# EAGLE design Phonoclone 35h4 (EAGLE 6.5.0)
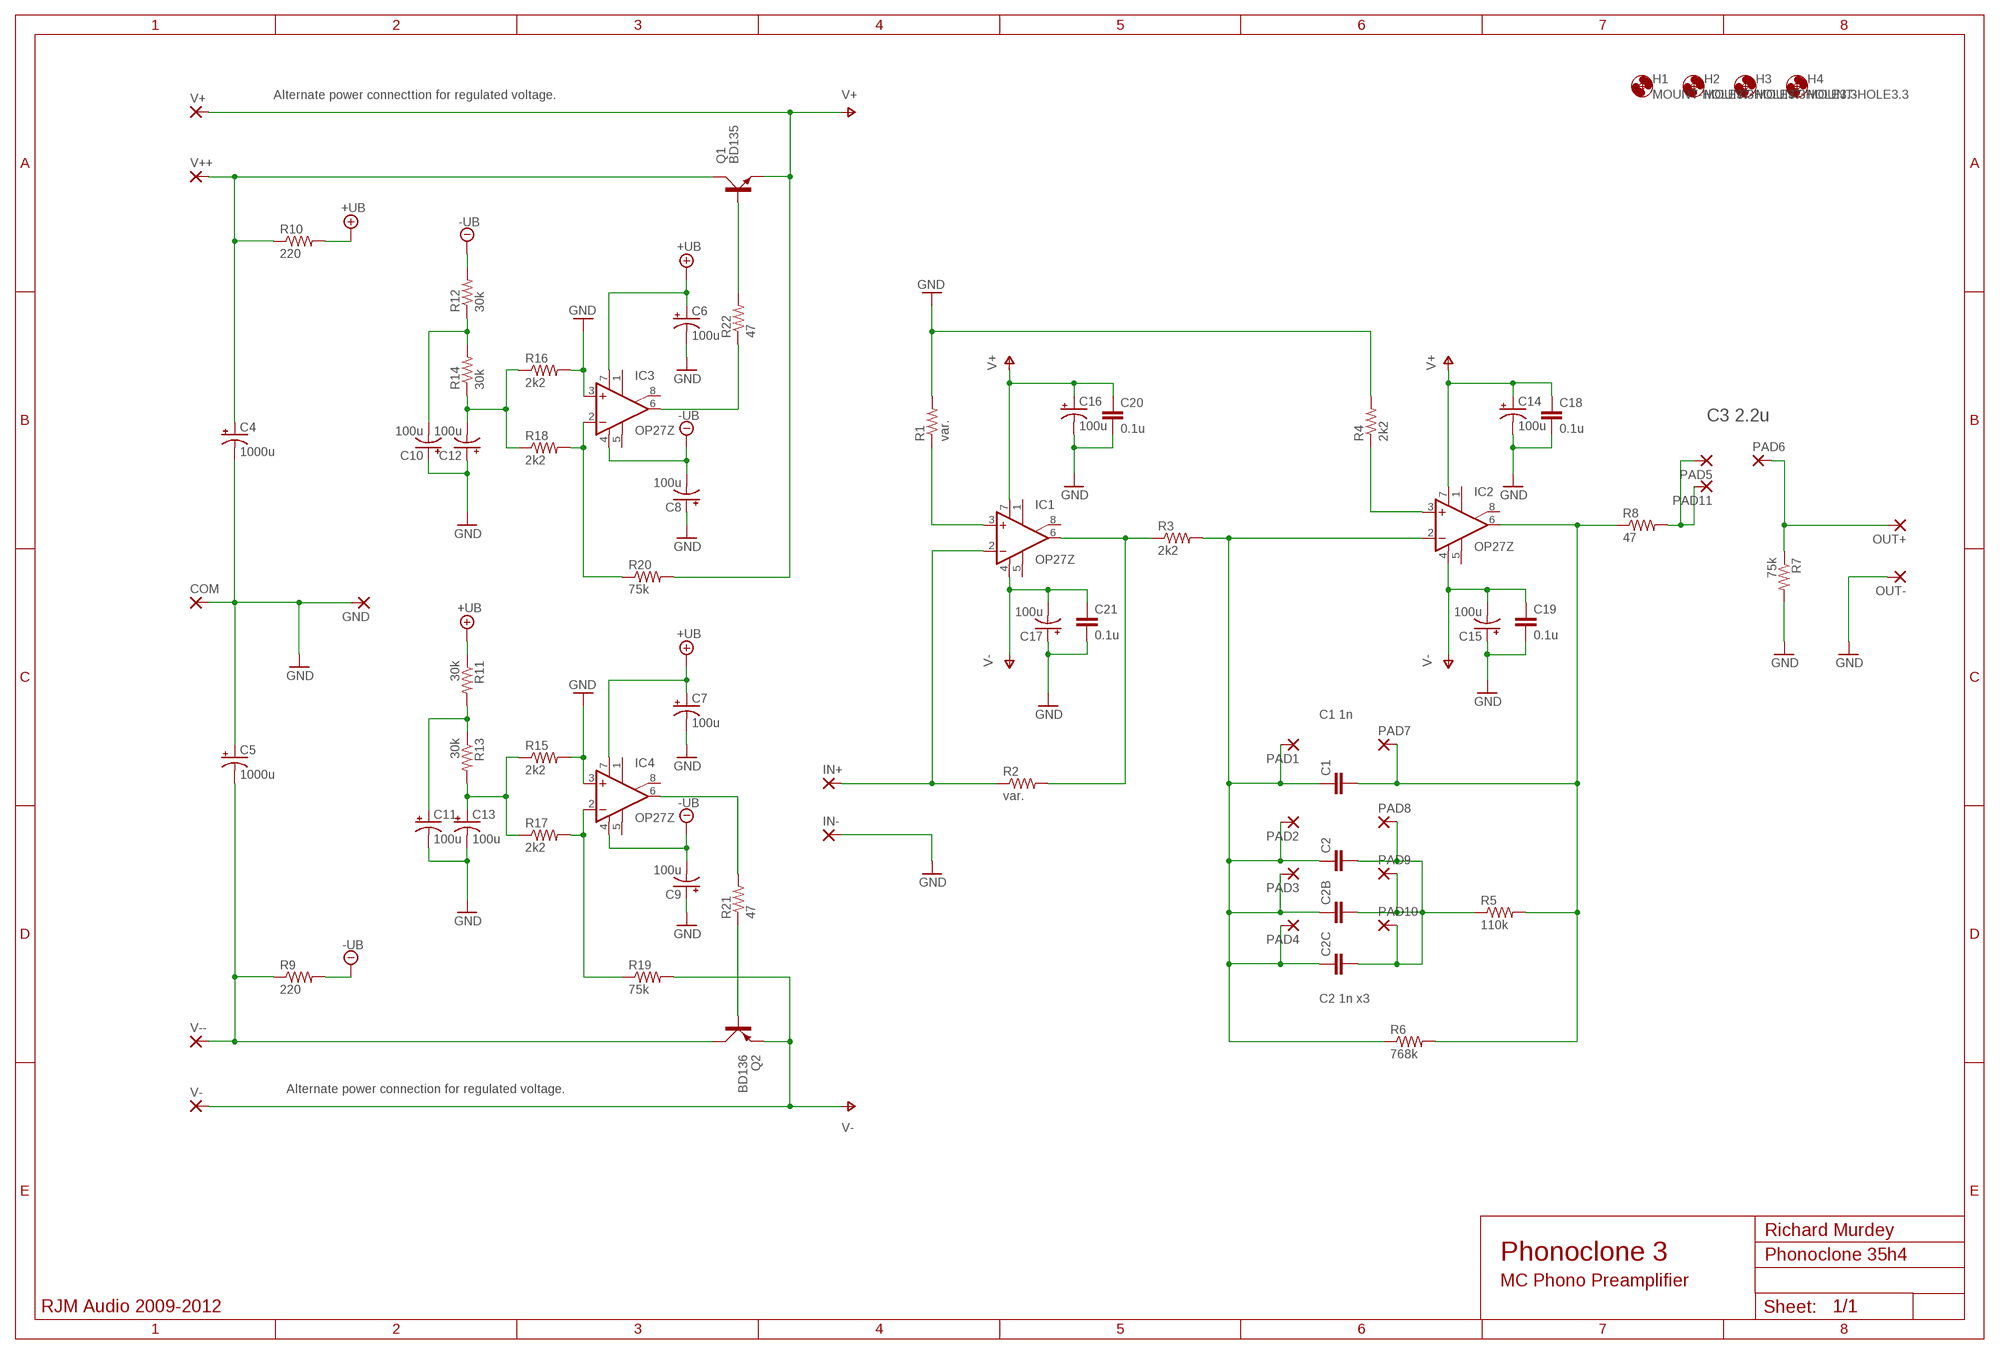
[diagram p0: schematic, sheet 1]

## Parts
C1  C5/4.5  [C5B4.5]
C2  C5/4.5  [C5B4.5]
C2B  C5/4.5  [C5B4.5]
C2C  C5/4.5  [C5B4.5]
C4  1000u  CPOL-USE5-10.5  [E5-10,5]
C5  1000u  CPOL-USE5-10.5  [E5-10,5]
C6  100u  CPOL-USE2.5-6  [E2,5-6]
C7  100u  CPOL-USE2.5-6  [E2,5-6]
C8  100u  CPOL-USE2.5-6  [E2,5-6]
C9  100u  CPOL-USE2.5-6  [E2,5-6]
C10  100u  CPOL-USE2.5-6  [E2,5-6]
C11  100u  CPOL-USE2.5-6  [E2,5-6]
C12  100u  CPOL-USE2.5-6  [E2,5-6]
C13  100u  CPOL-USE2.5-6  [E2,5-6]
C14  100u  CPOL-USE2.5-6  [E2,5-6]
C15  100u  CPOL-USE2.5-6  [E2,5-6]
C16  100u  CPOL-USE2.5-6  [E2,5-6]
C17  100u  CPOL-USE2.5-6  [E2,5-6]
C18  0.1u  C-EU050-024X044  [C050-024X044]
C19  0.1u  C-EU050-024X044  [C050-024X044]
C20  0.1u  C-EU050-024X044  [C050-024X044]
C21  0.1u  C-EU050-024X044  [C050-024X044]
COM  3,17/1,3  [3,17/1,3]
GND  3,17/1,3  [3,17/1,3]
H1  MOUNT-HOLE3.3  [3,3]
H2  MOUNT-HOLE3.3  [3,3]
H3  MOUNT-HOLE3.3  [3,3]
H4  MOUNT-HOLE3.3  [3,3]
IC1  OP27Z  [DIL08]
IC2  OP27Z  [DIL08]
IC3  OP27Z  [DIL08]
IC4  OP27Z  [DIL08]
IN+  2,54/1,1  [2,54/1,1]
IN-  2,54/1,1  [2,54/1,1]
OUT+  2,54/1,1  [2,54/1,1]
OUT-  2,54/1,1  [2,54/1,1]
PAD1  2,54/1,1  [2,54/1,1]
PAD2  2,54/1,1  [2,54/1,1]
PAD3  2,54/1,1  [2,54/1,1]
PAD4  2,54/1,1  [2,54/1,1]
PAD5  2,54/1,1  [2,54/1,1]
PAD6  2,54/1,1  [2,54/1,1]
PAD7  2,54/1,1  [2,54/1,1]
PAD8  2,54/1,1  [2,54/1,1]
PAD9  2,54/1,1  [2,54/1,1]
PAD10  2,54/1,1  [2,54/1,1]
PAD11  2,54/1,1  [2,54/1,1]
Q1  BD135  BD139  [TO126AV]
Q2  BD136  BD140  [TO126AV]
R1  var.  R-US_0207/10  [0207/10]
R2  var.  R-US_0207/10  [0207/10]
R3  2k2  R-US_0207/10  [0207/10]
R4  2k2  R-US_0207/10  [0207/10]
R5  110k  R-US_0207/10  [0207/10]
R6  768k  R-US_0207/10  [0207/10]
R7  75k  R-US_0207/10  [0207/10]
R8  47  R-US_0207/10  [0207/10]
R9  220  R-US_0207/10  [0207/10]
R10  220  R-US_0207/10  [0207/10]
R11  30k  R-US_0207/10  [0207/10]
R12  30k  R-US_0207/10  [0207/10]
R13  30k  R-US_0207/10  [0207/10]
R14  30k  R-US_0207/10  [0207/10]
R15  2k2  R-US_0207/10  [0207/10]
R16  2k2  R-US_0207/10  [0207/10]
R17  2k2  R-US_0207/10  [0207/10]
R18  2k2  R-US_0207/10  [0207/10]
R19  75k  R-US_0207/10  [0207/10]
R20  75k  R-US_0207/10  [0207/10]
R21  47  R-US_0207/10  [0207/10]
R22  47  R-US_0207/10  [0207/10]
V+  3,17/1,3  [3,17/1,3]
V++  3,17/1,3  [3,17/1,3]
V-  3,17/1,3  [3,17/1,3]
V--  3,17/1,3  [3,17/1,3]

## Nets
+UB: C6.+ C7.+ IC3.7(V+) IC4.7(V+) R10.2 R11.1
-UB: C8.- C9.- IC3.4(V-) IC4.4(V-) R9.2 R12.2
GND: C4.- C5.+ C6.- C7.- C8.+ C9.+ C10.+ C11.- C12.+ C13.- C14.- C15.+ C16.- C17.+ C18.2 C19.2 C20.2 C21.2 COM.1(P) GND.1(P) IC3.3(+IN) IC4.3(+IN) IN-.1(P) OUT-.1(P) R1.2 R4.2 R7.2 R15.2 R16.2
IN: IC1.2(-IN) IN+.1(P) R2.1
N$1: PAD5.1(P) PAD11.1(P) R8.2
N$4: C11.+ R11.2 R13.1
N$6: IC3.6(OUT) R22.1
N$7: Q1.B R22.2
N$8: IC1.3(+IN) R1.1
N$9: IC4.2(-IN) R17.2 R19.1
N$10: Q2.B R21.1
N$11: IC4.6(OUT) R21.2
N$13: IC3.2(-IN) R18.2 R20.1
N$14: C10.- R12.1 R14.2
OUT: IC1.6(OUT) R2.2 R3.1
OUT1: C1.2 IC2.6(OUT) PAD7.1(P) R5.2 R6.2 R8.1
OUT2: OUT+.1(P) PAD6.1(P) R7.1
P2+: IC2.3(+IN) R4.1
RIAA1: C1.1 C2.1 C2B.1 C2C.1 IC2.2(-IN) PAD1.1(P) PAD2.1(P) PAD3.1(P) PAD4.1(P) R3.2 R6.1
RIAA2: C2.2 C2B.2 C2C.2 PAD8.1(P) PAD9.1(P) PAD10.1(P) R5.1
V+: C14.+ C16.+ C18.1 C20.1 IC1.7(V+) IC2.7(V+) Q1.E R20.2 V+.1(P)
V++: C4.+ Q1.C R10.1 V++.1(P)
V-: C15.- C17.- C19.1 C21.1 IC1.4(V-) IC2.4(V-) Q2.E R19.2 V-.1(P)
V--: C5.- Q2.C R9.1 V--.1(P)
VREF+: C13.+ R13.2 R15.1 R17.1
VREF-: C12.- R14.1 R16.1 R18.1
Unconnected: IC1.1(ON1) IC1.5(OPT) IC1.8(ON2) IC2.1(ON1) IC2.5(OPT) IC2.8(ON2) IC3.1(ON1) IC3.5(OPT) IC3.8(ON2) IC4.1(ON1) IC4.5(OPT) IC4.8(ON2)

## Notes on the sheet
- Alternate power connecttion for regulated voltage.
- C3 2.2u
- C1 1n
- C2 1n x3
- Alternate power connection for regulated voltage.
- Richard Murdey
- Phonoclone 3
- MC Phono Preamplifier
- RJM Audio 2009-2012

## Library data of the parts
C1 C2 C2B C2C = capacitor-wima:C: CAPACITOR
C4-C17 = rcl:CPOL-US: POLARIZED CAPACITOR, American symbol
C18-C21 = resistor:C-EU: CAPACITOR, European symbol
COM GND V+ V++ V- V-- = wirepad:3,17/1,3: THROUGH-HOLE PAD
H1-H4 = holes:MOUNT-HOLE: MOUNTING HOLE with drill center marker
IC1-IC4 = linear:OP27: OP AMP
IN+ IN- OUT+ OUT- PAD1-PAD11 = wirepad:2,54/1,1: THROUGH-HOLE PAD
Q1 = transistor-power:BD139: NPN TRANSISTOR
Q2 = transistor-power:BD140: PNP TRANSISTOR
R1-R22 = rcl:R-US_: RESISTOR, American symbol

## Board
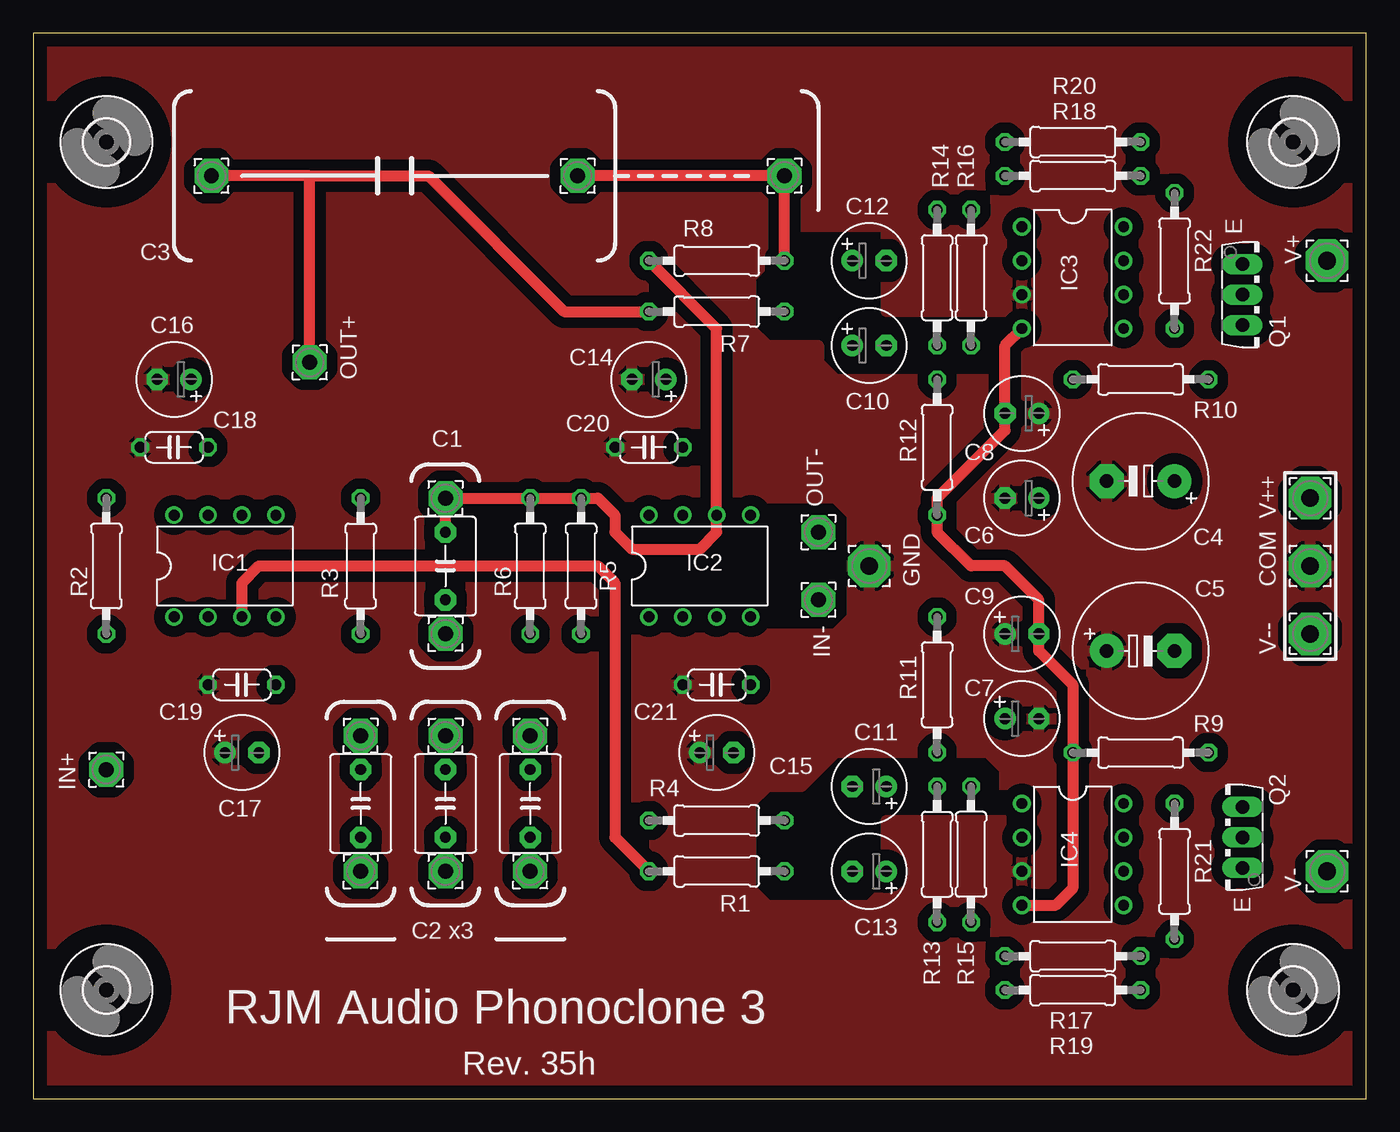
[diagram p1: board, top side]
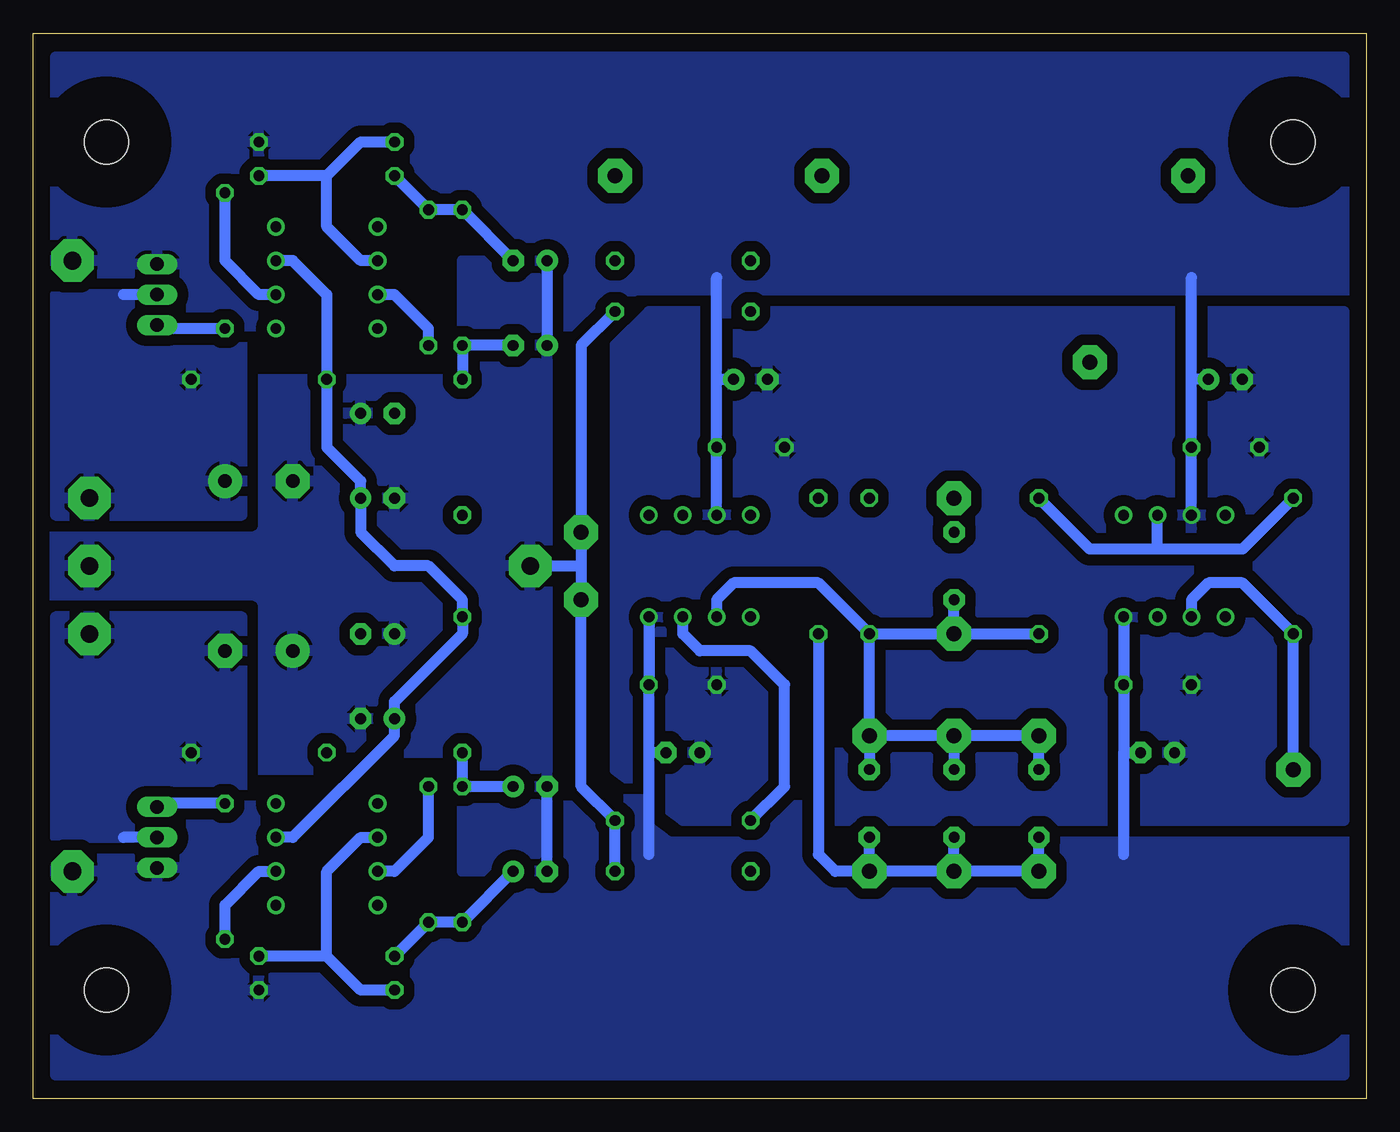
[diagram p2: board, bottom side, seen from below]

Size 99.82 x 79.76 mm. Coordinates in mm from the lower left corner, seen from the top.
Outline: 0,0 99.82,0 99.82,79.76 0,79.76 0,0
Copper layers (1*16): Top 0.035mm / dielectric 1.5mm / Bottom 0.035mm
Design rules "default": minimum track width 10mil, minimum drill 24mil, track to track 8mil, track to pad 8mil, pad to pad 8mil, via to via 8mil, smd to smd 8mil, copper to edge 40mil, drill to drill 8mil, minimum pad ring 10mil, minimum via ring 8mil, stop-mask expansion 4mil, vias tented up to drill 0mil, thermal gap 10mil

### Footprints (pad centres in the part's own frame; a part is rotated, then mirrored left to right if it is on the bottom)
C5B4.5 = drill 0.813 pad 1.6 octagon: 1 -2.54,0; 2 2.54,0
E5-10,5 = drill 1.016 pad 2.54: + -2.54,0 | drill 1.016 pad 2.54 octagon: - 2.54,0
E2,5-6 = drill 0.813 pad 1.6: + -1.27,0 | drill 0.813 pad 1.6 octagon: - 1.27,0
C050-024X044 = drill 0.813 octagon: 1 -2.54,0; 2 2.54,0
3,17/1,3 = drill 1.321 pad 3.175 octagon: 1 0,0
3,3 = hole 3.3: 0,0
DIL08 = drill 0.813 pad 1.27: 1 -3.81,-3.81; 2 -1.27,-3.81; 3 1.27,-3.81; 4 3.81,-3.81; 5 3.81,3.81; 6 1.27,3.81; 7 -1.27,3.81; 8 -3.81,3.81
2,54/1,1 = drill 1.118 pad 2.54 octagon: 1 0,0
TO126AV = drill 1.016 long: B 2.286,-1.27; C 0,-1.27; E -2.286,-1.27
0207/10 = drill 0.813 octagon: 1 -5.08,0; 2 5.08,0

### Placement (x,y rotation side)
C1  30.86,39.88 90 top
C2  24.51,22.1 270 top
C2B  30.86,22.1 270 top
C2C  37.21,22.1 270 top
C4  82.93,46.23 180 top
C5  82.93,33.53 0 top
C6  74.04,44.96 180 top
C7  74.04,28.45 0 top
C8  74.04,51.31 180 top
C9  74.04,34.8 0 top
C10  62.61,56.39 0 top
C11  62.61,23.37 180 top
C12  62.61,62.74 0 top
C13  62.61,17.02 180 top
C14  46.1,53.85 180 top
C15  51.18,25.91 0 top
C16  10.54,53.85 180 top
C17  15.62,25.91 0 top
C18  10.54,48.77 180 top
C19  15.62,30.99 180 top
C20  46.1,48.77 180 top
C21  51.18,30.99 180 top
COM  95.63,39.88 0 top
GND  62.61,39.88 0 top
H1  5.46,8.13 0 top
H2  5.46,71.63 0 top
H3  94.36,71.63 0 top
H4  94.36,8.13 0 top
IC1  14.35,39.88 0 top
IC2  49.91,39.88 0 top
IC3  77.85,61.47 270 top
IC4  77.85,18.29 270 top
IN+  5.46,24.64 0 top
IN-  58.8,37.34 0 top
OUT+  20.7,55.12 0 top
OUT-  58.8,42.42 0 top
PAD1  24.51,27.18 0 top
PAD2  30.86,27.18 0 top
PAD3  37.21,27.18 0 top
PAD4  30.86,34.8 0 top
PAD5  40.77,69.09 0 top
PAD6  13.34,69.09 0 top
PAD7  30.86,44.96 0 top
PAD8  24.51,17.02 0 top
PAD9  30.86,17.02 0 top
PAD10  37.21,17.02 0 top
PAD11  56.26,69.09 0 top
Q1  91.82,60.2 270 top
Q2  89.28,19.56 90 top
R1  51.18,17.02 0 top
R2  5.46,39.88 90 top
R3  24.51,39.88 270 top
R4  51.18,20.83 0 top
R5  41.02,39.88 90 top
R6  37.21,39.88 90 top
R7  51.18,58.93 0 top
R8  51.18,62.74 0 top
R9  82.93,25.91 180 top
R10  82.93,53.85 180 top
R11  67.69,30.99 270 top
R12  67.69,48.77 270 top
R13  67.69,18.29 270 top
R14  67.69,61.47 270 top
R15  70.23,18.29 90 top
R16  70.23,61.47 270 top
R17  77.85,10.67 0 top
R18  77.85,69.09 0 top
R19  77.85,8.13 0 top
R20  77.85,71.63 0 top
R21  85.47,17.02 270 top
R22  85.47,62.74 270 top
V+  96.9,62.74 90 top
V++  95.63,44.96 0 top
V-  96.9,17.02 90 top
V--  95.63,34.8 0 top

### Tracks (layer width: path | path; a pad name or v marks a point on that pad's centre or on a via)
+UB
  Bottom 0.813: IC3.7 80.39,62.74 77.85,60.2 R10.2 77.85,48.77 75.31,46.23 C6.+ 75.31,42.42 72.77,39.88 70.23,39.88 67.69,37.34 R11.1 67.69,34.8 72.77,29.72 C7.+ 72.77,27.18 80.39,19.56 IC4.7
-UB
  Top 0.813: IC3.4 72.77,56.39 C8.- 72.77,50.04 67.69,44.96 R12.2 67.69,42.42 70.23,39.88 72.77,39.88 75.31,37.34 C9.- 75.31,33.53 77.85,30.99 R9.2 77.85,15.75 76.58,14.48 IC4.4
GND
  Bottom 0.813: R7.2 58.8,56.39 OUT-.1 58.8,39.88 | R15.2 70.23,19.56 72.77,17.02 IC4.3 | R16.2 70.23,57.66 72.77,60.2 IC3.3 | R1.2 R4.2 58.8,23.37 IN-.1 58.8,39.88 | GND.1 58.8,39.88 | C12.+ C10.+ | C13.- C11.-
  pour Top (isolate 0.813): 0.38,79.25 72.77,79.25 72.77,58.93 63.88,58.93 63.88,65.28 57.53,65.28 53.72,61.47 53.72,15.75 54.99,14.48 62.61,14.48 63.88,15.75 63.88,20.83 72.77,20.83 72.77,0.51 0.38,0.51
  pour Bottom (isolate 0.813, rank 3): 98.17,44.96 82.93,44.96 82.93,53.85 67.69,53.85 67.69,62.74 61.34,62.74 61.34,17.02 67.69,17.02 67.69,25.91 72.77,25.91 72.77,24.64 82.93,24.64 82.93,34.8 98.17,34.8
  pour Top (isolate 0.813): 72.77,79.25 99.44,79.25 99.44,0.51 72.77,0.51
  pour Top (isolate 0.813): 53.72,44.96 53.72,57.66 54.99,56.39 58.8,56.39 58.8,55.12 60.07,53.85 72.77,53.85 72.77,24.64 71.5,25.91 60.07,25.91 57.53,23.37 54.99,23.37 53.72,22.1 53.72,34.8 60.07,34.8 61.34,36.07 61.34,43.69 60.07,44.96
  pour Bottom (isolate 0.813): 1.65,58.93 53.72,58.93 56.26,56.39 56.26,24.64 51.18,20.83 1.65,20.83
IN
  Bottom 0.813: IN+.1 R2.1 9.27,38.61 11.81,38.61 13.08,37.34 IC1.2
N$1
  Top 0.813: PAD5.1 PAD11.1 R8.2
N$4
  Bottom 0.813: C11.+ R13.1 R11.2
N$6
  Bottom 0.813: IC3.6 82.93,60.2 85.47,62.74 R22.1
N$7
  Bottom 0.813: R22.2 90.3,57.66 Q1.B
N$8
  Top 0.813: IC1.3 15.62,38.61 16.89,39.88 42.29,39.88 43.56,38.61 43.56,19.56 R1.1
N$9
  Bottom 0.813: R19.1 75.31,8.13 77.85,10.67 | 77.85,10.67 R17.2 | IC4.2 75.31,19.56 77.85,17.02 77.85,10.67
N$10
  Bottom 0.813: R21.1 90.3,22.1 Q2.B
N$11
  Bottom 0.813: IC4.6 82.93,17.02 85.47,14.48 R21.2
N$13
  Bottom 0.813: 77.85,69.09 75.31,71.63 R20.1 | 77.85,69.09 R18.2 | IC3.2 75.31,62.74 77.85,65.28 77.85,69.09
N$14
  Bottom 0.813: C10.- R14.2 R12.1
OUT
  Bottom 0.813: R2.2 9.27,41.15 15.62,41.15 | 15.62,41.15 IC1.6 | 15.62,41.15 20.7,41.15 R3.1
OUT1
  Top 0.813: R8.1 51.18,57.66 IC2.6 51.18,42.42 49.91,41.15 44.83,41.15 43.56,42.42 43.56,43.69 42.29,44.96 R5.2 R6.2 PAD7.1 C1.2
OUT2
  Top 0.813: 20.7,69.09 PAD6.1 | OUT+.1 20.7,69.09 | R7.1 39.75,58.93 29.59,69.09 20.7,69.09
P2+
  Bottom 0.813: IC2.3 51.18,34.8 49.91,33.53 46.1,33.53 43.56,30.99 43.56,23.37 R4.1
RIAA1
  Bottom 0.813: PAD4.1 C1.1 | PAD4.1 R3.2 | R6.1 PAD4.1 | R6.1 41.02,38.61 47.37,38.61 48.64,37.34 IC2.2 | PAD2.1 PAD1.1 C2.1 | PAD2.1 PAD3.1 | PAD2.1 C2B.1 | PAD3.1 C2C.1 | PAD3.1 R6.1
RIAA2
  Bottom 0.813: PAD9.1 PAD8.1 C2.2 | PAD9.1 PAD10.1 | PAD9.1 C2B.2 | PAD10.1 C2C.2 | PAD10.1 39.75,17.02 41.02,18.29 R5.1
V+
  Bottom 0.813: C16.+ 13.08,53.85 | 13.08,53.85 13.08,61.47 | 48.64,53.85 48.64,61.47 | IC1.7 C18.1 13.08,53.85 | IC2.7 C20.1 48.64,53.85 | 48.64,53.85 C14.+
  pour Bottom (isolate 0.813, rank 4): 1.65,41.15 1.65,77.98 98.17,77.98 98.17,41.15
V++
  Bottom 0.813: Q1.C 93.09,60.2
  pour Bottom (isolate 0.813): 98.17,43.69 84.2,43.69 84.2,57.66 90.55,57.66 90.55,60.2 98.17,60.2
V-
  Bottom 0.813: 18.16,18.29 18.16,25.91 | 18.16,25.91 C17.- | 53.72,18.29 53.72,25.91 | 53.72,25.91 C21.1 IC2.4 | IC1.4 C19.1 18.16,25.91 | C15.- 53.72,25.91
  pour Bottom (isolate 0.813, rank 4): 1.65,1.78 1.65,38.61 67.69,38.61 98.17,38.61 98.17,1.78
V--
  Bottom 0.813: Q2.C 93.09,19.56
  pour Bottom (isolate 0.813): 84.2,36.07 98.17,36.07 98.17,19.56 90.55,19.56 90.55,22.1 84.2,22.1
VREF+
  Bottom 0.813: C13.+ R13.2 R15.1 R17.1
VREF-
  Bottom 0.813: C12.- R14.1 R16.1 R18.1

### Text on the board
tPlace: C3 | C2 x3 | RJM Audio Phonoclone 3 | Rev. 35h
tNames: E | E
